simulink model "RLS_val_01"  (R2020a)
settings: Solver=ode45  StartTime=0.0  StopTime=1000  RelTol=1e-3  EnableMultiTasking=on
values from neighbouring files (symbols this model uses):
  Ts = 0.05    [init_model.m]
libraries: ctrlSharedLib x2

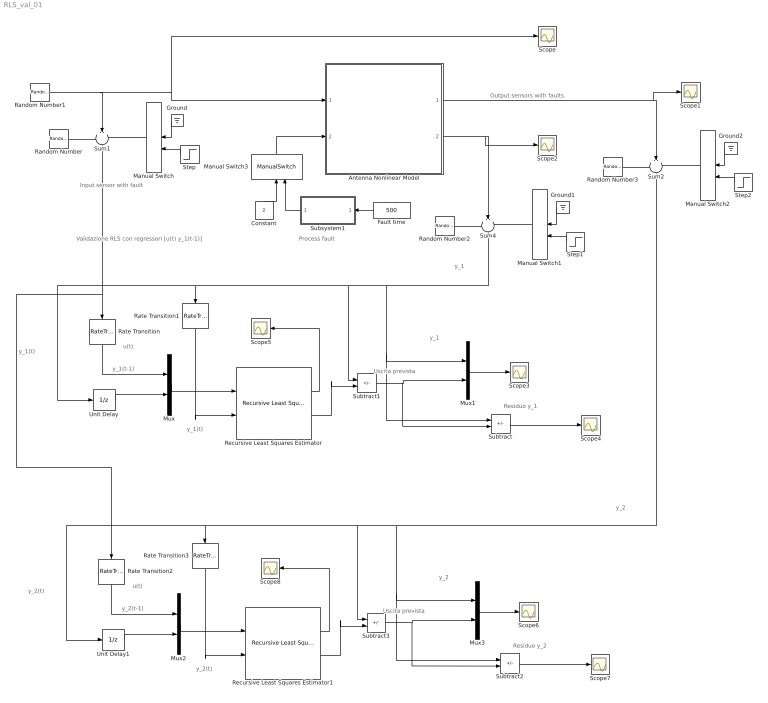
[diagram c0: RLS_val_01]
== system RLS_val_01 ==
  note: Residuo y_1
  note: Uscita prevista
  note: Validazione RLS con regressori [u(t) y_1(t-1)]
  note: y_1(t)
  note: y_1(t-1)
  note: y_1
  note: u(t)
  note: Output sensors with faults
  note: Process fault
  note: Input sensor with fault
  note: y_1(t)
  note: y_1
  note: y_2(t)
  note: y_2
  note: y_2
  note: y_2(t-1)
  note: u(t)
  note: y_2(t)
  note: Residuo y_2
  note: Uscita prevista
  Antenna Nonlinear Model : Subsystem
  Constant : Constant  Value=2
  Fault time : Constant  Value=500
  Ground : Ground
  Ground1 : Ground
  Ground2 : Ground
  Manual Switch : ManualSwitch
  Manual Switch1 : ManualSwitch
  Manual Switch2 : ManualSwitch
  Manual Switch3 : ManualSwitch  CurrentSetting=0
  Mux{,1..3} (4 alike) : Mux  Inputs=2
  Random Number : RandomNumber  Variance=0.0001  Seed=1  SampleTime=Ts
  Random Number1 : RandomNumber  Variance=0.1  SampleTime=10
  Random Number2 : RandomNumber  Variance=0.00001  Seed=2  SampleTime=Ts
  Random Number3 : RandomNumber  Variance=0.00001  Seed=3  SampleTime=Ts
  Rate Transition{,1..3} (4 alike) : RateTransition  OutPortSampleTime=Ts
  Recursive Least Squares Estimator : ctrlSharedLib/Recursive Least Squares Estimator  InitialEstimateSource=None  InitialParameterData=2  P0=1e4  InitialRegressors=0  InitialOutputs=0  History=Infinite  WindowLength=200  EstimationMethod=Forgetting Factor  AdaptationParameter=1  HasTimeVaryingAdaptationParameter=off  NormalizationBias=eps  OutputError=on  OutputP=off  AddEnablePort=off  InputProcessing=Sample-based  Ts=Ts
  Recursive Least Squares Estimator1 : ctrlSharedLib/Recursive Least Squares Estimator  InitialEstimateSource=None  InitialParameterData=2  P0=1e4  InitialRegressors=0  InitialOutputs=0  History=Infinite  WindowLength=200  EstimationMethod=Forgetting Factor  AdaptationParameter=1  HasTimeVaryingAdaptationParameter=off  NormalizationBias=eps  OutputError=on  OutputP=off  AddEnablePort=off  InputProcessing=Sample-based  Ts=Ts
  Scope{,1..8} (9 alike) : Scope
  Step : Step  Time=500  SampleTime=0
  Step1 : Step  Time=500  SampleTime=0
  Step2 : Step  Time=500  SampleTime=0
  Subsystem1 : Subsystem
  Subtract{,1..3} (4 alike) : Sum  Inputs=+-
  Sum1 : Sum  Inputs=+++  SaturateOnIntegerOverflow=on
  Sum2 : Sum  Inputs=+++  SaturateOnIntegerOverflow=on
  Sum4 : Sum  Inputs=+++  SaturateOnIntegerOverflow=on
  Unit Delay : UnitDelay  SampleTime=Ts  HasFrameUpgradeWarning=on
  Unit Delay1 : UnitDelay  SampleTime=Ts  HasFrameUpgradeWarning=on
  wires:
  Random Number1/1 -> Scope/1, Antenna Nonlinear Model/1(force), Sum1/2
  Random Number/1 -> Sum1/1
  Manual Switch/1 -> Sum1/3
  Ground/1 -> Manual Switch/1
  Step/1 -> Manual Switch/2
  Random Number2/1 -> Sum4/1
  Ground1/1 -> Manual Switch1/1
  Manual Switch1/1 -> Sum4/3
  Step1/1 -> Manual Switch1/2
  Antenna Nonlinear Model/2(velocity) -> Sum4/2, Scope2/1
  Random Number3/1 -> Sum2/1
  Ground2/1 -> Manual Switch2/1
  Manual Switch2/1 -> Sum2/3
  Step2/1 -> Manual Switch2/2
  Antenna Nonlinear Model/1(angle) -> Sum2/2, Scope1/1
  Fault time/1 -> Subsystem1/1(Fault time)
  Subsystem1/1(Fault) -> Manual Switch3/2
  Manual Switch3/1 -> Antenna Nonlinear Model/2(drag)
  Constant/1 -> Manual Switch3/1
  Mux/1 -> Recursive Least Squares Estimator/1
  Sum4/1 -> Subtract/1, Mux1/1, Subtract1/1, Rate Transition1/1, Unit Delay/1
  Unit Delay/1 -> Mux/2
  Subtract1/1 -> Subtract/2, Mux1/2
  Mux1/1 -> Scope3/1
  Subtract/1 -> Scope4/1
  Rate Transition/1 -> Mux/1
  Rate Transition1/1 -> Recursive Least Squares Estimator/2
  Recursive Least Squares Estimator/2 -> Subtract1/2
  Recursive Least Squares Estimator/1 -> Scope5/1
  Recursive Least Squares Estimator1/2 -> Subtract3/2
  Rate Transition2/1 -> Mux2/1
  Mux3/1 -> Scope6/1
  Recursive Least Squares Estimator1/1 -> Scope8/1
  Unit Delay1/1 -> Mux2/2
  Subtract2/1 -> Scope7/1
  Sum1/1 -> Rate Transition2/1, Rate Transition/1
  Sum2/1 -> Subtract2/1, Mux3/1, Subtract3/1, Rate Transition3/1, Unit Delay1/1
  Subtract3/1 -> Subtract2/2, Mux3/2
  Rate Transition3/1 -> Recursive Least Squares Estimator1/2
  Mux2/1 -> Recursive Least Squares Estimator1/1

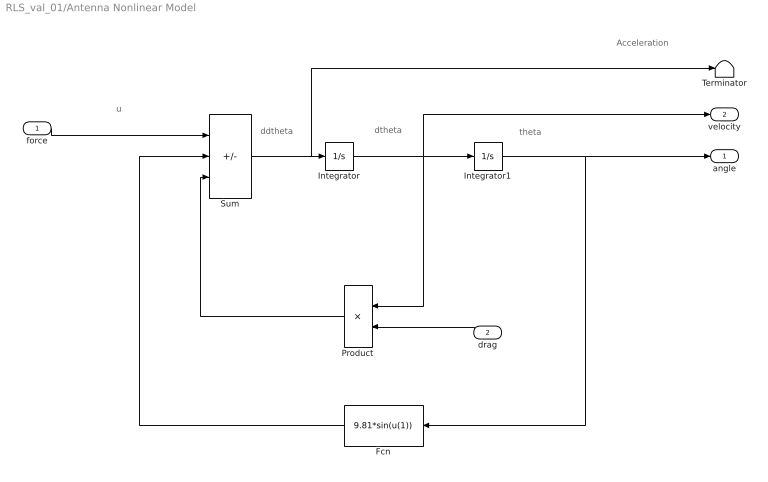
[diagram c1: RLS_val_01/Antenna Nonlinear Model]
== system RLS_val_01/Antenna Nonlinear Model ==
  note: Acceleration
  note: ddtheta
  note: dtheta
  note: theta
  note: u
  force : Inport
  drag : Inport  Port=2
  Fcn : Fcn  Expr=9.81*sin(u(1))
  Integrator : Integrator
  Integrator1 : Integrator  InitialCondition=(pi/180)*90
  Product : Product
  Sum : Sum  Inputs=+--  SaturateOnIntegerOverflow=on
  Terminator : Terminator
  angle : Outport
  velocity : Outport  Port=2
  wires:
  Sum/1 -> Terminator/1, Integrator/1
  Integrator/1 -> Product/1, Integrator1/1, velocity/1
  Integrator1/1 -> angle/1, Fcn/1
  Fcn/1 -> Sum/2
  Product/1 -> Sum/3
  force/1 -> Sum/1
  drag/1 -> Product/2

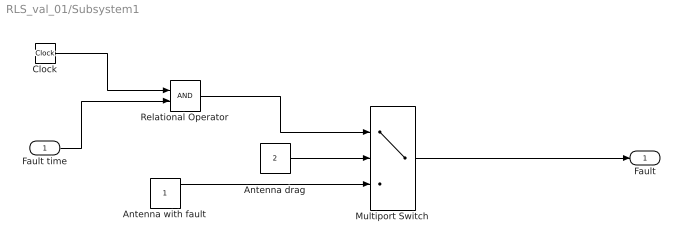
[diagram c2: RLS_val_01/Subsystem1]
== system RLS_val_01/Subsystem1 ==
  Fault time : Inport
  Antenna drag : Constant  Value=2
  Antenna with fault : Constant
  Clock : Clock
  Multiport Switch : MultiPortSwitch  DataPortOrder=Zero-based contiguous  Inputs=2  zeroidx=on
  Relational Operator : RelationalOperator  OutDataTypeStr=boolean  RndMeth=Simplest
  Fault : Outport
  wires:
  Clock/1 -> Relational Operator/1
  Fault time/1 -> Relational Operator/2
  Antenna drag/1 -> Multiport Switch/2
  Relational Operator/1 -> Multiport Switch/1
  Multiport Switch/1 -> Fault/1
  Antenna with fault/1 -> Multiport Switch/3
